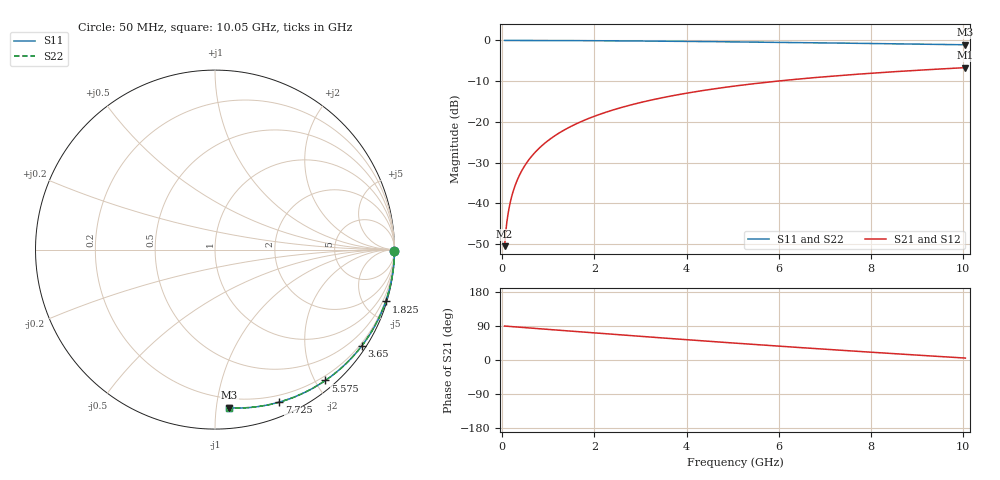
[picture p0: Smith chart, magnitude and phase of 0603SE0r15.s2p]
! AVX Thin Film Operation		Date: August 2001
! Description: Accu-P® Series, Thin Film, SMD, RF Capacitor
! Part Number: 06035J0R15ABT
! 50 MHz  -  10.05 GHz
! Serial Measurements
# mhz S db R 50
!	S11		S21		S12		S22
!	dB	Phase	dB	Phase	dB	Phase	dB	Phase
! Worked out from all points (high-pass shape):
!   401 points, 50 MHz to 10.05 GHz, reference 50 ohm
!   highest |S21| = -6.67 dB at 10.05 GHz (marker M1); lowest = -50.5 dB at 50 MHz (marker M2)
!   |S21| within 3 dB of the highest: 6.249 GHz to end of sweep
!   lowest |S11| = -1.1 dB at 10.05 GHz (marker M3), VSWR 16.39, Z = 6.67 - j54.3 ohm
!   |S11| at or under -10 dB: nowhere
!   |S22| runs from -1.1 to 0.0 dB; largest |S21 - S12| = 0
!   S11 on the Smith chart (normalised r, x): 50 MHz: open; 1.825 GHz: 0.14, -6.73; 3.65 GHz: 0.13, -3.34; 5.575 GHz: 0.13, -2.14; 7.725 GHz: 0.13, -1.50; 10.05 GHz: 0.13, -1.09
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50  -0.00 -0.5  -50.51 89.6  -50.51 89.6  -0.00 -0.5
75  -0.00 -0.7  -46.99 89.4  -46.99 89.4  -0.00 -0.7
125  -0.00 -1.2  -42.56 88.9  -42.56 88.9  -0.00 -1.2
150  -0.00 -1.4  -40.97 88.6  -40.97 88.6  -0.00 -1.4
225  -0.00 -2.1  -37.45 87.9  -37.45 87.9  -0.00 -2.1
275  -0.00 -2.6  -35.71 87.5  -35.71 87.5  -0.00 -2.6
350  -0.00 -3.3  -33.62 86.7  -33.62 86.7  -0.00 -3.3
500  -0.00 -4.6  -30.52 85.4  -30.52 85.4  -0.00 -4.6
725  -0.01 -6.7  -27.30 83.3  -27.30 83.3  -0.01 -6.7
1000  -0.01 -9.3  -24.53 80.7  -24.53 80.7  -0.01 -9.3
1325  -0.03 -12.3  -22.11 77.7  -22.11 77.7  -0.03 -12.3
1725  -0.04 -16.0  -19.85 74.0  -19.85 74.0  -0.04 -16.0
1825  -0.05 -16.9  -19.38 73.1  -19.38 73.1  -0.05 -16.9
2525  -0.10 -23.3  -16.65 66.7  -16.65 66.7  -0.10 -23.3
3400  -0.17 -31.1  -14.23 58.9  -14.23 58.9  -0.17 -31.1
3650  -0.19 -33.3  -13.66 56.6  -13.66 56.6  -0.19 -33.3
5050  -0.35 -45.5  -11.18 44.5  -11.18 44.5  -0.35 -45.4
5575  -0.41 -49.9  -10.47 40.1  -10.47 40.1  -0.41 -49.9
6725  -0.56 -59.3  -9.18 30.7  -9.18 30.7  -0.56 -59.3
7725  -0.70 -67.2  -8.28 22.7  -8.28 22.7  -0.70 -67.2
8400  -0.80 -72.4  -7.75 17.5  -7.75 17.5  -0.80 -72.4
10050  -1.06 -84.8  -6.67 5.1  -6.67 5.1  -1.06 -84.8
